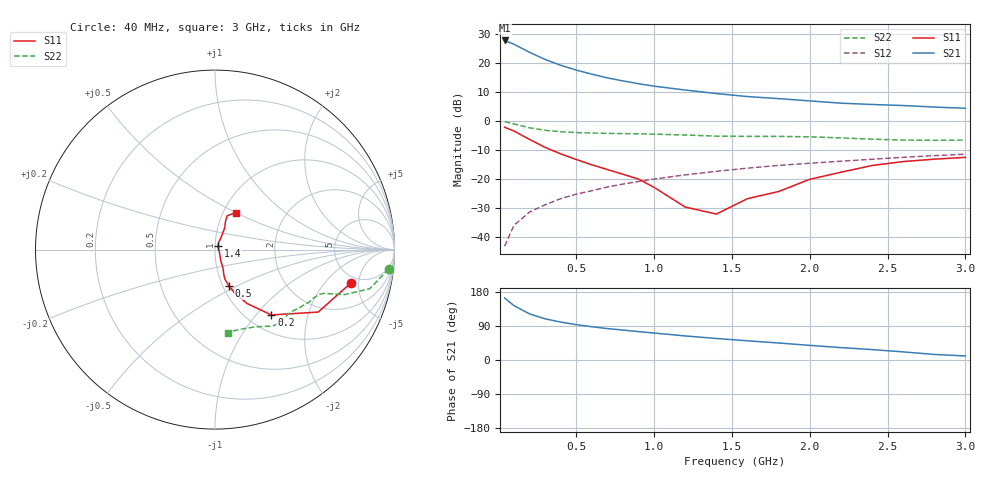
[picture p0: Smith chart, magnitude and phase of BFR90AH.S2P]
! Filename:  BFR90AH.S2P  Version:  2.0
! Philips part #: BFR90A  Date: Jul 1990
! Bias condition: Vce=10V,  Ic=10mA
#  MHz  S  MA  R  50
! Freq  S11  S21  S12  S22  !GUM [dB]
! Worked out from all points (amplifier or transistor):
!   21 points, 40 MHz to 3 GHz, reference 50 ohm
!   highest |S21| = 27.7 dB at 40 MHz (marker M1)
!   |S21| within 3 dB of that: start of sweep to 161 MHz
!   unconditionally stable (mu >= 1): 713.3 MHz to end of sweep
!   at 300 MHz: K = 0.82, MSG = 25.0 dB, |S12| = -28.9 dB
!   at 1 GHz: K = 1.04, MAG = 14.8 dB, |S12| = -20.0 dB
!   at 3 GHz: K = 1.01, MAG = 7.3 dB, |S12| = -11.4 dB
!   S11 on the Smith chart (normalised r, x): 40 MHz: 4.16, -3.96; 200 MHz: 1.28, -1.21; 500 MHz: 1.07, -0.45; 1.4 GHz: 1.03, +0.04; 3 GHz: 1.15, +0.50
40  0.779 -13.9  24.29 163.6  0.007 82.5  0.974 -6.4
100  0.672 -31.2  20.89 143.5  0.016 74.2  0.889 -14.2
200  0.481 -49.2  15.18 121.7  0.027 69.8  0.763 -19.2
300  0.351 -59.1  11.46 108.7  0.036 68.7  0.69 -20.9
400  0.272 -65.2  9.092 100.1  0.046 68.7  0.653 -21.9
500  0.217 -68.9  7.51 93.3  0.055 68.6  0.631 -23.4
600  0.176 -71.4  6.391 87.8  0.063 68.1  0.62 -24.9
700  0.146 -70.5  5.514 82.9  0.073 67.5  0.611 -26.2
800  0.121 -67.6  4.885 79.0  0.082 66.7  0.606 -27.6
900  0.1 -65.5  4.373 74.9  0.091 65.5  0.601 -28.9
1000  0.072 -63.1  3.967 71.2  0.1 64.3  0.593 -30.3
1200  0.033 -38.7  3.408 63.5  0.118 61.3  0.573 -34.2
1400  0.025 47.3  2.963 56.8  0.136 58.1  0.548 -39.1
1600  0.046 62.7  2.629 50.6  0.154 56.0  0.542 -44.3
1800  0.061 62.7  2.422 44.9  0.172 53.3  0.542 -49.3
2000  0.099 64.7  2.214 38.6  0.187 49.9  0.533 -53.1
2200  0.131 65.8  2.023 32.7  0.203 47.1  0.511 -56.8
2400  0.171 69.8  1.922 27.5  0.219 44.1  0.486 -62.3
2600  0.2 70.2  1.843 21.4  0.237 40.5  0.469 -69.7
2800  0.22 64.5  1.735 14.7  0.253 37.3  0.464 -76.6
3000  0.236 60.5  1.653 10.7  0.268 35.1  0.469 -81.2
